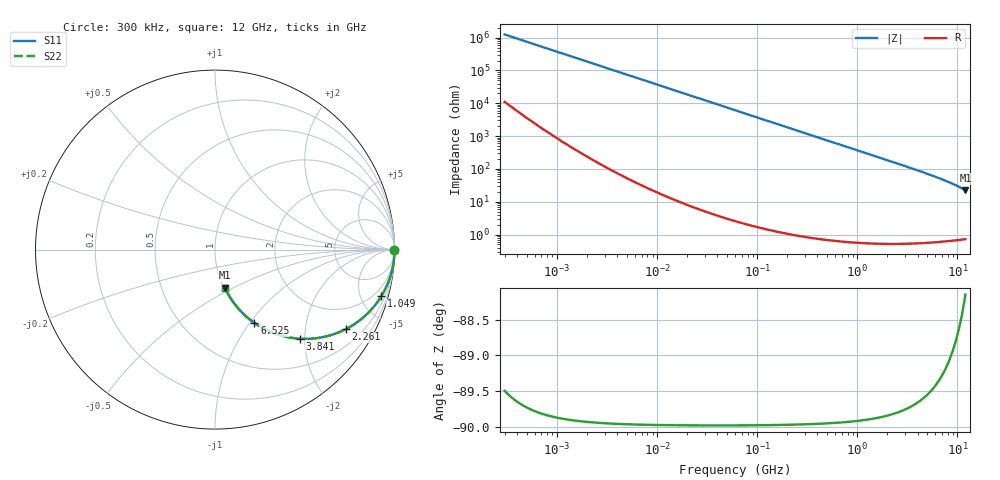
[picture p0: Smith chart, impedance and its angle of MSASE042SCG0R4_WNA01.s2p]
! MSASE042SCG0R4_WNA01  S-PARAMETER MODEL  ( General Type )
! Model Generated by TAIYO YUDEN Corporation (http://www.ty-top.com)
! Version 1.0
! TAIYO YUDEN Control No. 130801
! Copyright(c) 2013 TAIYO YUDEN CO.,LTD. All Rights Reserved.
! Product Description (link to TY-COMPAS)
! https://ds.yuden.co.jp/TYCOMPAS/or/detail?pn=MSASE042SCG0R4AWNA01&u=M
! Products Name : Multilayer Ceramic Capacitors
! Characteristics :
!  Capacitance : 0.4 pF , Rated Voltage : 16V , TCC : CG / C0G
!  Case Size : 0.4 x 0.2 / 0.016 x 0.008 [mm/inch] , Thickness : 0.2 / 0.008 [mm/inch]
!  (Conditions: Temperature = 25 degC , DC Bias Current/Voltage = 0A / 0V)
! External Node Assignments :
!  1  o---| |---o  2
! GND o---------o GND
! Frequency Range : 0.3MHz  -  12000MHz  [ 401 STEP ]
# MHz S RI R 50
! Freq[MHz].  S11 Real  S11 Imag  S21 Real  S21 Imag  S12 Real  S12 Imag  S22 Real  S22 Imag
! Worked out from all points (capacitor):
!   401 points, 300 kHz to 12 GHz, reference 50 ohm
!   read as one part in series: C = 425 fF near 316.3 kHz
!   lowest |Z| = 22.5 ohm at 12 GHz (marker M1)
!   S11 on the Smith chart (normalised r, x): 300 kHz: open; 1.049 GHz: 1.01, -7.12; 2.261 GHz: 1.01, -3.28; 3.841 GHz: 1.01, -1.89; 6.525 GHz: 1.01, -1.05; 12 GHz: 1.01, -0.45
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0.3  1 -8.02e-05  7.15e-07 8.02e-05  7.15e-07 8.02e-05  1 -8.02e-05
0.361125  1 -9.65e-05  6.85e-07 9.65e-05  6.85e-07 9.65e-05  1 -9.65e-05
0.390996  1 -0.000105  6.75e-07 0.000105  6.75e-07 0.000105  1 -0.000105
1.769972  1 -0.000473  8.83e-07 0.000473  8.83e-07 0.000473  1 -0.000473
10.44266  1 -0.00279  9.2e-06 0.00279  9.2e-06 0.00279  1 -0.00279
60  0.9997 -0.016  0.000264 0.016  0.000264 0.016  0.9997 -0.016
164.1901  0.9981 -0.0438  0.00195 0.0438  0.00195 0.0438  0.9981 -0.0438
353.9943  0.9911 -0.0938  0.00895 0.0938  0.00895 0.0938  0.9911 -0.0938
617.4538  0.9733 -0.1607  0.0267 0.1607  0.0267 0.1607  0.9733 -0.1607
826.3444  0.9531 -0.2107  0.0469 0.2107  0.0469 0.2107  0.9531 -0.2107
1048.836  0.9265 -0.2602  0.0735 0.2602  0.0735 0.2602  0.9265 -0.2602
1262.535  0.8968 -0.3034  0.1032 0.3034  0.1032 0.3034  0.8968 -0.3034
1519.776  0.8567 -0.3493  0.1433 0.3493  0.1433 0.3493  0.8567 -0.3493
2088.533  0.7587 -0.4264  0.2413 0.4264  0.2413 0.4264  0.7587 -0.4264
2261.293  0.7279 -0.4435  0.2721 0.4435  0.2721 0.4435  0.7279 -0.4435
3026.31  0.5955 -0.4886  0.4045 0.4886  0.4045 0.4886  0.5955 -0.4886
3841.137  0.4726 -0.4964  0.5274 0.4964  0.5274 0.4964  0.4726 -0.4964
4875.354  0.3501 -0.4732  0.6499 0.4732  0.6499 0.4732  0.3501 -0.4732
6524.734  0.2196 -0.4083  0.7804 0.4083  0.7804 0.4083  0.2196 -0.4083
7648.807  0.162 -0.3614  0.838 0.3614  0.838 0.3614  0.162 -0.3614
8966.534  0.1151 -0.31  0.8849 0.31  0.8849 0.31  0.1151 -0.31
12000  0.0545 -0.2114  0.9455 0.2114  0.9455 0.2114  0.0545 -0.2114
